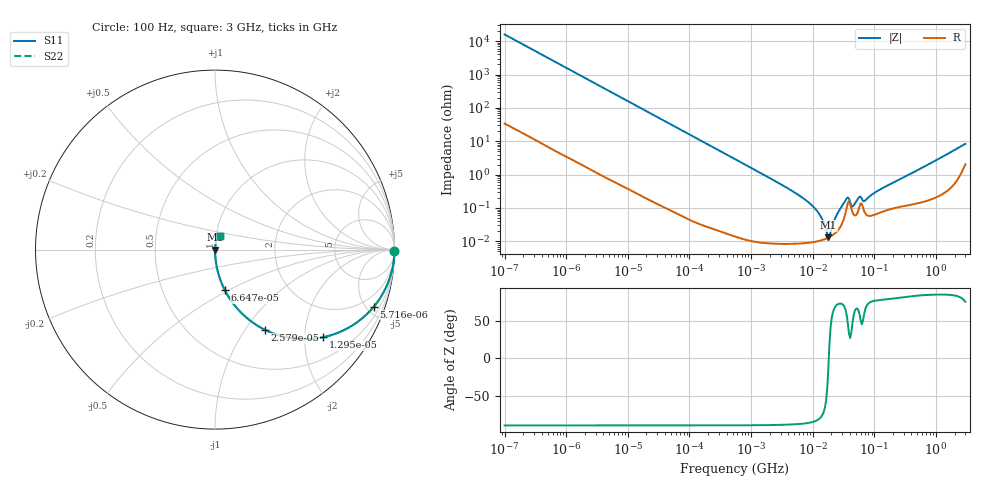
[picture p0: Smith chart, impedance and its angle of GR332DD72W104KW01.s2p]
!Murata Part Number: GR332DD72W104KW01
!These Parameters are Measured in Series Mode Connection
!Data Generated on Jun 19, 2026
!  o--ll--o
!Port1  Port2
!  o------o
!Operation Temp=25[degC], DC Bias Voltage=0[V]
!Freq. Start=100[Hz] Stop=3[GHz] 401[Steps]
# Hz S RI R 50
!Freq.(Hz) S11(Real) S11(Imag) S21(Real) S21(Imag) S12(Real) S12(Imag) S22(Real) S22(Imag)
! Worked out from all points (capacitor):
!   401 points, 100 Hz to 3 GHz, reference 50 ohm
!   read as one part in series: C = 101 nF near 109 Hz
!   lowest |Z| = 13.4 mohm at 17.89 MHz (marker M1)
!   series resonance near 18.21 MHz, so ESL is about 760 pH
!   S11 on the Smith chart (normalised r, x): 100 Hz: open; 5.716 kHz: 1.01, -5.57; 12.95 kHz: 1.01, -2.46; 25.79 kHz: 1.00, -1.24; 66.47 kHz: 1.00, -0.48; 3 GHz: 1.04, +0.16
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100  0.9999 -0.00632  5.34e-05 0.00632  5.34e-05 0.00632  0.9999 -0.00632
1788  0.9873 -0.111  0.0127 0.111  0.0127 0.111  0.9873 -0.111
5716  0.8852 -0.3176  0.1148 0.3176  0.1148 0.3176  0.8852 -0.3176
12951  0.6022 -0.4883  0.3978 0.4883  0.3978 0.4883  0.6022 -0.4883
25785  0.2774 -0.4465  0.7226 0.4465  0.7226 0.4465  0.2774 -0.4465
31977  0.2001 -0.3988  0.7999 0.3988  0.7999 0.3988  0.2001 -0.3988
66468  0.0552 -0.227  0.9448 0.227  0.9448 0.227  0.0552 -0.227
164120  0.00971 -0.0965  0.9903 0.0965  0.9903 0.0965  0.00971 -0.0965
547723  0.000994 -0.0292  0.999 0.0292  0.999 0.0292  0.000994 -0.0292
4323298  9.66e-05 -0.00351  0.9999 0.00351  0.9999 0.00351  9.66e-05 -0.00351
9794414  9.54e-05 -0.00118  0.9999 0.00118  0.9999 0.00118  9.54e-05 -0.00118
1.323817e7  0.000106 -0.000585  0.9999 0.000585  0.9999 0.000585  0.000106 -0.000585
1.713898e7  0.000125 -0.000111  0.9999 0.000111  0.9999 0.000111  0.000125 -0.000111
1.789277e7  0.00013 -3.23e-05  0.9999 3.23e-05  0.9999 3.23e-05  0.00013 -3.23e-05
1.950129e7  0.000141 0.000128  0.9999 -0.000128  0.9999 -0.000128  0.000141 0.000128
2.52476e7  0.000208 0.000658  0.9998 -0.000658  0.9998 -0.000658  0.000208 0.000658
3.562563e7  0.00105 0.00165  0.999 -0.00165  0.999 -0.00165  0.00105 0.00165
4.612319e7  0.000637 0.00101  0.9994 -0.00101  0.9994 -0.00101  0.000637 0.00101
5.719833e7  0.00108 0.00186  0.9989 -0.00186  0.9989 -0.00186  0.00108 0.00186
7.093284e7  0.000699 0.00153  0.9993 -0.00153  0.9993 -0.00153  0.000699 0.00153
1.751444e8  0.000927 0.00495  0.9991 -0.00495  0.9991 -0.00495  0.000927 0.00495
3e9  0.026 0.0774  0.974 -0.0774  0.974 -0.0774  0.026 0.0774
